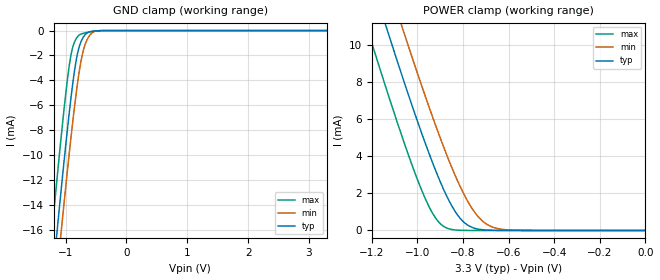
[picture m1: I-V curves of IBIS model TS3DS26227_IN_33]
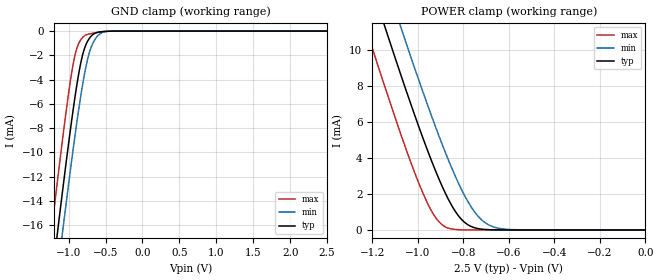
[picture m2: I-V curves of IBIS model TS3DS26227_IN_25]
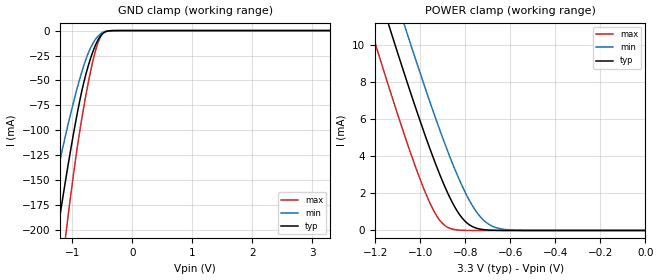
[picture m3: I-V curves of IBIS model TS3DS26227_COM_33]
| TEXAS INSTRUMENTS INCORPORATED
| Standard Linear and Logic Group
| IBIS Model of TS3DS26227
| 7 Ohm Dual SPDT Differential Signal Switch
| With Input Logic Translation
| This file contains package information for the following:
|  TVSOP 14-pin (DGV) package as [Component] TS3DS26227_DGV
| This device can be powered at the following Vccs:
|  3.3 volt Vcc
|  2.5 volt Vcc
| This file provides unique models under the [Model Selector] for each Vcc.
| For operation at a specific Vcc, select the appropriate model after each
| [Model Selector] keyword.
[IBIS Ver]   3.2
[Comment char]  |_char
[File Name]   ts3ds26227.ibs
[File Rev]   1.1 | x_die
[Date]   May 11, 2006
[Source]   Data created from TI-SPICE simulations at TI-SLL.
[Notes]   The following is an IBIS list for the TS3DS26227.
   Please contact sllibis@ti.com with questions and
   comments concerning SLL IBIS models.
   - FILE REV HISTORY
   - 1.1 Release IBIS file on 05/17/06
   - Non-monotonic data due to FET characteristics.
   - 14-pin (DGV) package parasitics were used. Actual package
   12-pin (YZP/YZT) parasitics should be better.
[Disclaimer] Property of Texas Instruments Incorporated.  Unauthorized
   reproduction and/or distribution is strictly prohibited.
   This product is protected under copyright law.
   Created  2006, (C) Copyright  2006, Texas Instruments
   Incorporated, All Rights Reserved
   UNLESS THERE IS A SIGNED, WRITTEN AGREEMENT TO THE
   CONTRARY, TEXAS INSTRUMENTS (TI) IS PROVIDING THE IBIS
   MODELS  AND WITHOUT ANY WARRANTY, EXPRESSED OR
   IMPLIED.  TI assumes no liability for:
   1) the accuracy of the IBIS models provided to your
   company;
   2) the proper functioning of these IBIS Models in your
   design or for any resulting applications; or
   3) infringement of patents, copyrights or intellectual
   property rights resulting from your use of these IBIS
   models.
   TI provides IBIS Models as a service to our customers.
   You and your company shall not distribute, sell or give
   these models to anyone else without prior written
   permission from TI.
   TI reserves the right to make changes to our products or
   to discontinue any semiconductor product or service
   without notice, and advises our customers to obtain the
   latest version of relevant information to verify, before
   placing orders, that the information being relied on is
   current.
   Please be aware that your receipt and use of the IBIS
   information provided shall serve as acceptance of these
   terms and conditions.  If you do not accept these terms,
   you should return or destroy the IBIS models and any
   other accompanying information immediately.
| Component TS3DS26227_DGV 14-PIN TVSOP
[Component]   TS3DS26227_DGV
[Manufacturer]   Texas Instruments, Inc.
[Package]
|   typ   min   max
R_pkg   3.500e-02   2.000e-02   4.500e-02
L_pkg   2.499e-09   2.077e-09   2.966e-09
C_pkg   3.610e-13   3.050e-13   4.160e-13
[Pin]   signal_name   model_name   R_pin   L_pin   C_pin
1   IN2   TS3DS26227_IN   2.700e-02   2.717e-09   3.730e-13
2   VIO   POWER   3.700e-02   2.434e-09   3.980e-13
3   IN1   TS3DS26227_IN   3.400e-02   2.200e-09   3.160e-13
4   NC1   TS3DS26227_NX   2.000e-02   2.077e-09   3.090e-13
5   GND   GND   3.000e-02   2.147e-09   3.050e-13
6   NC2   TS3DS26227_NX   4.200e-02   2.580e-09   4.080e-13
7   COM2   TS3DS26227_COM   3.900e-02   2.921e-09   3.850e-13
8   GND   GND   3.300e-02   2.841e-09   3.800e-13
9   COM1   TS3DS26227_COM   4.200e-02   2.611e-09   4.100e-13
10   NO1   TS3DS26227_NX   3.800e-02   2.331e-09   3.290e-13
11   V+   POWER   2.600e-02   2.223e-09   3.190e-13
12   NO2   TS3DS26227_NX   3.400e-02   2.259e-09   3.130e-13
13   NC   NC   4.500e-02   2.681e-09   4.160e-13
14   NC   NC   4.200e-02   2.966e-09   3.860e-13
[Series Switch Groups]
| Function Group States
On  1 /   | COM1->NC1 IN1 LOW
On  2 /   | COM2->NC2 IN2 LOW
On  3 /   | COM1->NO1 IN1 HIGH
On  4 /   | COM2->NO2 IN2 HIGH
On  5 /   | NC1->COM1 IN1 LOW
On  6 /   | NC2->COM2 IN2 LOW
On  7 /   | NO1->COM1 IN1 HIGH
On  8 /   | NO2->COM2 IN2 HIGH
Off 1 5 /   | IN1 HIGH
Off 2 6 /   | IN2 HIGH
Off 3 7 /   | IN1 LOW
Off 4 8 /   | IN2 LOW
[Series Pin Mapping]   pin_2   model_name   function_table_group
9   4   TS3DS26227_COM_33_S   1
| 9   4   TS3DS26227_COM_25_S   1
7   6   TS3DS26227_COM_33_S   2
| 7   6   TS3DS26227_COM_25_S   2
9   10   TS3DS26227_COM_33_S   3
| 9   10   TS3DS26227_COM_25_S   3
7   12   TS3DS26227_COM_33_S   4
| 7   12   TS3DS26227_COM_25_S   4
4   9   TS3DS26227_NX_33_S   5
| 4   9   TS3DS26227_NX_25_S   5
6   7   TS3DS26227_NX_33_S   6
| 6   7   TS3DS26227_NX_25_S   6
10   9   TS3DS26227_NX_33_S   7
| 10   9   TS3DS26227_NX_25_S   7
12   7   TS3DS26227_NX_33_S   8
| 12   7   TS3DS26227_NX_25_S   8
| Model TS3DS26227_IN
[Model Selector]   TS3DS26227_IN
TS3DS26227_IN_33   3.3 volt Vcc
TS3DS26227_IN_25   2.5 volt Vcc
| Model TS3DS26227_COM
[Model Selector]   TS3DS26227_COM
TS3DS26227_COM_33   3.3 volt Vcc
TS3DS26227_COM_25   2.5 volt Vcc
| Model TS3DS26227_COM_S
[Model Selector]   TS3DS26227_COM_S
TS3DS26227_COM_33_S   3.3 volt Vcc
TS3DS26227_COM_25_S   2.5 volt Vcc
| Model TS3DS26227_NX
[Model Selector]   TS3DS26227_NX
TS3DS26227_NX_33   3.3 volt Vcc
TS3DS26227_NX_25   2.5 volt Vcc
| Model TS3DS26227_NX_S
[Model Selector]   TS3DS26227_NX_S
TS3DS26227_NX_33_S   3.3 volt Vcc
TS3DS26227_NX_25_S   2.5 volt Vcc
[Model]   TS3DS26227_COM_33_S
Model_type  Series_switch
| variable   typ   min   max
C_comp   0   0   0
[Temperature Range]   40   100   -40
| Ambient temperature   25   85   -40
[Voltage range]   3.3   3   3.6
[On]
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[Off]
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[Model]   TS3DS26227_COM_25_S
Model_type  Series_switch
| variable   typ   min   max
C_comp   0   0   0
[Temperature Range]   40   100   -40
| Ambient temperature   25   85   -40
[Voltage range]   2.5   2.3   2.7
[On]
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[Off]
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[Model]   TS3DS26227_NX_33_S
Model_type  Series_switch
| variable   typ   min   max
C_comp   0   0   0
[Temperature Range]   40   100   -40
| Ambient temperature   25   85   -40
[Voltage range]   3.3   3   3.6
[On]
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[Off]
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[Model]   TS3DS26227_NX_25_S
Model_type  Series_switch
| variable   typ   min   max
C_comp   0   0   0
[Temperature Range]   40   100   -40
| Ambient temperature   25   85   -40
[Voltage range]   2.5   2.3   2.7
[On]
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[Off]
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| Models and submodels in the file (10): TS3DS26227_IN_33 (Input), TS3DS26227_IN_25 (Input), TS3DS26227_COM_33_S (Series_switch), TS3DS26227_COM_33 (Terminator), TS3DS26227_COM_25_S (Series_switch), TS3DS26227_COM_25 (Terminator), TS3DS26227_NX_33_S (Series_switch), TS3DS26227_NX_33 (Terminator), TS3DS26227_NX_25_S (Series_switch), TS3DS26227_NX_25 (Terminator)
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[Model]   TS3DS26227_IN_33
Model_type  Input
Vinl=0.5775
Vinh=1.2675
| variable   typ   min   max
C_comp   1.35pF   1.23pF   1.59pF
[Temperature Range]   40   100   -40
| Ambient temperature   25   85   -40
[Voltage range]   3.3   3   3.6
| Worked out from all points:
|   GND clamp passes 1 mA (typ) near -0.76 V on its own axis
|   POWER clamp passes 1 mA (typ) near -0.83 V on its own axis
[GND Clamp]
| TS3DS26227_IN_33
|   Voltage   I(typ)   I(min)   I(max)
-3.3V     -132.5mA   -134.9mA   -129.5mA
-1.23V    -20.63mA   -23.99mA   -16.4mA
-1.145V   -16.32mA   -19.7mA    -12.05mA
-1.075V   -12.85mA   -16.23mA   -8.587mA
-985mV    -8.566mA   -11.9mA    -4.489mA
-915mV    -5.502mA   -8.691mA   -2.025mA
-835mV    -2.624mA   -5.343mA   -719.8uA
-760mV    -1.047mA   -2.789mA   -307.6uA
-710mV    -527.7uA   -1.608mA   -221.5uA
-650mV    -200.4uA   -759.3uA   -151.4uA
-495mV    -24.11uA   -38.62uA   -24.75uA
3.3V      80.19pA    6.39nA     38.36pA
[POWER Clamp]
| TS3DS26227_IN_33
|   Voltage   I(typ)   I(min)   I(max)
-3.3V     101.2mA    103.7mA    98.32mA
-1.215V   14.04mA    16.7mA     10.7mA
-1.13V    10.72mA    13.38mA    7.394mA
-1.07V    8.447mA    11.09mA    5.157mA
-1.06V    8.074mA    10.71mA    4.796mA
-980mV    5.197mA    7.759mA    2.13mA
-910mV    2.924mA    5.324mA    501.7uA
-815mV    691.1uA    2.434mA    11.72uA
-760mV    165.2uA    1.179mA    1.001uA
-715mV    40.4uA     514uA      132.7nA
-600mV    889.2nA    27.96uA    809pA
-48.03fV  80.19pA    119.3pA    42.82pA
[Model]   TS3DS26227_IN_25
Model_type  Input
Vinl=0.5775
Vinh=1.2675
| variable   typ   min   max
C_comp   1.38pF   1.27pF   1.60pF
[Temperature Range]   40   100   -40
| Ambient temperature   25   85   -40
[Voltage range]   2.5   2.3   2.7
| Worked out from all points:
|   GND clamp passes 1 mA (typ) near -0.76 V on its own axis
|   POWER clamp passes 1 mA (typ) near -0.83 V on its own axis
[GND Clamp]
| TS3DS26227_IN_25
|   Voltage   I(typ)   I(min)   I(max)
-2.5V     -88.7mA    -91.44mA   -85.32mA
-1.235V   -20.89mA   -24.25mA   -16.66mA
-1.155V   -16.82mA   -20.2mA    -12.55mA
-1.135V   -15.82mA   -19.2mA    -11.54mA
-1.09V    -13.58mA   -16.97mA   -9.315mA
-1.07V    -12.6mA    -15.98mA   -8.346mA
-935mV    -6.342mA   -9.588mA   -2.616mA
-845mV    -2.927mA   -5.735mA   -816.5uA
-770mV    -1.19mA    -3.081mA   -335.4uA
-665mV    -257.2uA   -925.3uA   -167.9uA
-505mV    -28.06uA   -48.78uA   -29.66uA
2.5V      59.19pA    484.5pA    28.22pA
[POWER Clamp]
| TS3DS26227_IN_25
|   Voltage   I(typ)   I(min)   I(max)
-2.5V     67.33mA    69.82mA    64.3mA
-1.245V   15.22mA    17.89mA    11.89mA
-1.21V    13.84mA    16.5mA     10.5mA
-1.15V    11.49mA    14.15mA    8.16mA
-1.125V   10.53mA    13.19mA    7.204mA
-1.075V   8.634mA    11.28mA    5.339mA
-975mV    5.025mA    7.58mA     1.983mA
-910mV    2.924mA    5.324mA    501.7uA
-810mV    618.6uA    2.303mA    9.381uA
-710mV    34.34uA    462.1uA    106nA
-600mV    889.2nA    27.96uA    795.7pA
-31.15fV  59.19pA    102.9pA    30.89pA
[Model]   TS3DS26227_COM_33
Model_type  Terminator
| variable   typ   min   max
C_comp   8.93pF   6.68pF   10.81pF
| C_tri-state   8.93pF   6.68pF   10.81pF
[Temperature Range]   40   100   -40
| Ambient temperature   25   85   -40
[Voltage range]   3.3   3   3.6
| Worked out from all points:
|   GND clamp passes 1 mA (typ) near -0.44 V on its own axis
|   POWER clamp passes 1 mA (typ) near -0.83 V on its own axis
[GND Clamp]
| TS3DS26227_COM_33
|   Voltage   I(typ)   I(min)   I(max)
-3.3V     -1.171A    -906.7mA   -1.395A
-1.455V   -288.2mA   -204.7mA   -382.5mA
-1.415V   -271.3mA   -192.3mA   -361.4mA
-1.235V   -198mA     -139.1mA   -268.5mA
-1.095V   -144.7mA   -101mA     -199mA
-920mV    -84.51mA   -58.52mA   -119mA
-775mV    -44.54mA   -29.49mA   -66mA
-615mV    -15.09mA   -9.114mA   -20.99mA
-555mV    -7.836mA   -4.713mA   -9.831mA
-495mV    -3.173mA   -1.981mA   -3.278mA
-325mV    -57.72uA   -56.1uA    -22.07uA
3.3V      8.235nA    18.66nA    3.754nA
[POWER Clamp]
| TS3DS26227_COM_33
|   Voltage   I(typ)   I(min)   I(max)
-3.3V     101.2mA    103.7mA    98.32mA
-1.215V   14.04mA    16.7mA     10.7mA
-1.13V    10.72mA    13.38mA    7.394mA
-1.07V    8.447mA    11.09mA    5.157mA
-1.06V    8.074mA    10.71mA    4.796mA
-980mV    5.197mA    7.759mA    2.13mA
-910mV    2.924mA    5.324mA    501.7uA
-815mV    691.1uA    2.434mA    11.72uA
-760mV    165.2uA    1.179mA    1.005uA
-715mV    40.41uA    514.1uA    137nA
-600mV    898.7nA    27.98uA    5.041nA
-48.03fV  8.235nA    11.94nA    3.973nA
